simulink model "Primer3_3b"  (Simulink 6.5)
settings: Solver=ode23t  SolverMode=SingleTasking  StartTime=0.0  StopTime=1  RelTol=1e-3  AbsTol=1e-6
undefined symbols (not defined in the file or in its folder): Continuous, powergui, steady, ZData
libraries: powerlib x5, powerlib_extras x2

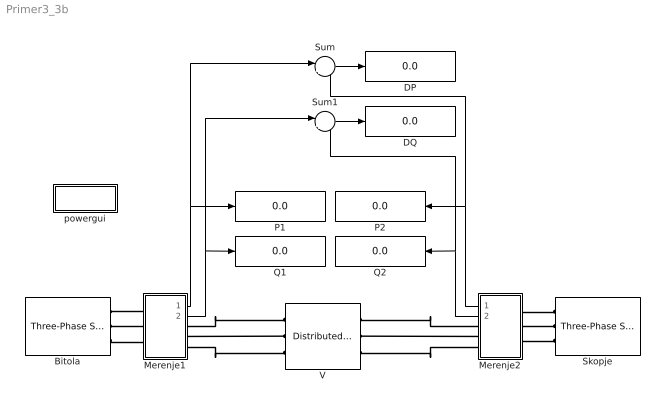
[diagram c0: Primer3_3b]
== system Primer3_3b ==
  Bitola : powerlib/Electrical Sources/Three-Phase Source  DialogController=PMDialogs.PMDefaultMaskDlg  SystemSampleTime=-1  Voltage=410e3  PhaseAngle=0  Frequency=50  InternalConnection=Yg  SpecifyImpedance=on  Resistance=0.8929  Inductance=16.58e-3  ShortCircuitLevel=sqrt(3)*400e3*16e3  BaseVoltage=400e3  XRratio=10
  DP : Display
  DQ : Display
  Merenje1 : Subsystem
  Merenje2 : Subsystem  Orientation=left
  P1 : Display
  P2 : Display
  Q1 : Display
  Q2 : Display
  Skopje : powerlib/Electrical Sources/Three-Phase Source  Orientation=left  DialogController=PMDialogs.PMDefaultMaskDlg  SystemSampleTime=-1  Voltage=395e3  PhaseAngle=-2.5  Frequency=50  InternalConnection=Yg  SpecifyImpedance=on  Resistance=0.8929  Inductance=16.58e-3  ShortCircuitLevel=sqrt(3)*400e3*14e3  BaseVoltage=400e3  XRratio=10
  Sum : Sum  Inputs=|++
  Sum1 : Sum  Inputs=|++
  V : powerlib/Elements/Distributed Parameters Line  DialogController=PMDialogs.PMDefaultMaskDlg  SystemSampleTime=-1  Phases=3  Frequency=50  Resistance=[0.029983 0.29405]  Inductance=[0.0010055 0.0025377]  Capacitance=[1.1784e-008 8.6541e-009]  Length=113.5  x1=[0 8.60953493752654e-011 155617.901806502 -377100.173822709;0.000106379256748321 8.65325079837872e-011 168131.358149619 -371689.815392539;0.000212758513496643 8.68730275722288e-011 180457.046333984 -365864.355859094;0.000319137770244964 8.7116527850222e-011 192581.201100092 -359630.30106294;0.000425517026993286 8.72627368780204e-011 204490.282259832 -352994.613161546;0.000531896283741607 8.7311491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  x2=[0 1.52828084545043e-010 143893.096531519 -373225.666404169;0.000106379256748321 1.57548911798779e-010 156283.637924653 -368209.241884694;0.000212758513496643 1.62093789310554e-010 168499.6426266 -362781.603346936;0.000319137770244964 1.66457641386629e-010 180527.467871754 -356948.812347202;0.000425517026993286 1.70635594501455e-010 192353.681052273 -350717.382913801;0.000531896283741607 1.7462298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  x3=[0 -7.90373299703389e-013 525.422105317868 -979.122392884629;0.000106379256748321 -7.55164225839465e-013 557.844919090553 -961.019300144194;0.000212758513496643 -7.19111788799262e-013 589.644734783168 -941.842946433889;0.000319137770244964 -6.82256251742466e-013 620.786038539719 -921.614747798094;0.000425517026993286 -6.44638774726363e-013 651.234051926655 -900.357294975707;0.000531896283741607 -6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  x4=[0 1.19047082254412e-012 334.073009196058 -1629.8040871509;0.000106379256748321 1.13114510037133e-012 388.344425208523 -1617.73135760439;0.000212758513496643 1.07055612168819e-012 442.182140342785 -1603.85195474176;0.000319137770244964 1.0087715519266e-012 495.52602894023 -1588.18137900235;0.000425517026993286 9.45860391747901e-013 548.316516844957 -1570.73713119736;0.000531896283741607 8.81892899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  x5=0.000531896283741607  Measurements=None
  powergui : Subsystem  AncestorBlock=powerlib/powergui  InitFcn=powergui( 'InitFcn_Callback' , gcb , 0 , [ ] );  mask(PSB option menu block){SimulationMode=Continuous, SampleTime=50e-6, echomessages=off, RestoreLinks=warning, x0status=steady, Frange=[0:2:500], Ylog=off, Xlog=on, ShowGrid=off, save=off, variable=ZData, structure=, ZoomFFT=on, StartTime=0.0, cycles=1, DisplayStyle=1, fundamental=60, FreqAxis=off, MaxFrequency=1000, frequencyindice=50, frequencyindicesteady=1, RmsSteady=2, display=off, Ts=0, frequency=60, methode=off, HookPort=off, Interpol=off}
      mask prompts: SimulationMode "Simulation mode"; SampleTime "Sample time Ts (when simulation mode is Discrete) (s)"; echomessages "Echo  Messages"; RestoreLinks "Restore disabled links"; x0status "Initial electrical states status"; Frange "Impedance tool: Frequency Range"; Ylog "Impedance tool: Log impedance"; Xlog "Impedance tool: log Frequency"; ShowGrid "Impedance tool: grid"; save "Impedance tool: Save Data To Workspace"; variable "Impedance tool: Variable Name"; structure "Structure Name (PSBFFTSCOPE)"; ZoomFFT "ZoomFFT (PSBFFTSCOPE)"; StartTime "Start Time (PSBFFTSCOPE)"; cycles "Cycles (PSBFFTSCOPE)"; DisplayStyle "Display style (PSBFFTSCOPE)"; fundamental "Fundamental (PSBFFTSCOPE)"; FreqAxis "Frequency Axis (PSBFFTSCOPE)"; MaxFrequency "Max Frequency (PSBFFTSCOPE)"; frequencyindice "Load flow frequency (Hz)"; frequencyindicesteady "Frequency indice (STEADYSTATE)"; RmsSteady "RMS display (STEADYSTATE)"; display "Display Results"; Ts "OBSOLETE 1"; frequency "Phasor frequency (Hz)"; methode "Phasor simulation"; HookPort "Hook port"; Interpol "Interpolate"
      mask init:
      | powerlibroot = which('powersysdomain');
      | PSBroot = powerlibroot(1:end-16);
      | %
      | switch SimulationMode
      | 	case 1
      | 		message=sprintf('Continuous');
      | 	case 2
      |         SampleTimeeval=evalin('base',SampleTime,'NaN');
      |         if isnan(SampleTimeeval)
      |             message=sprintf('Warning !!,\nUndefined sample time');
      |         else
      |             message=sprintf('Discrete,\nTs = %.4g s.',SampleTimeeval);
      |         end
      | 	case 3
      | 		message=sprintf('Phasors');
      | end
      | if strcmp(bdroot,'powerlib')
      |   message='powergui';
      | end
      | power_initmask();
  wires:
  Merenje1/1(P) -> P1/1, Sum/1
  Merenje1/2(Q) -> Q1/1, Sum1/1
  Merenje2/1(P) -> P2/1, Sum/2
  Merenje2/2(Q) -> Q2/1, Sum1/2
  Sum/1 -> DP/1
  Sum1/1 -> DQ/1
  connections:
  Bitola/RConn1 -- Merenje1/LConn1
  Bitola/RConn2 -- Merenje1/LConn2
  Bitola/RConn3 -- Merenje1/LConn3
  Merenje1/RConn2 -- V/LConn2
  Merenje1/RConn3 -- V/LConn3
  Merenje1/RConn1 -- V/LConn1
  Merenje2/LConn2 -- Skopje/RConn2
  Merenje2/LConn1 -- Skopje/RConn1
  Merenje2/LConn3 -- Skopje/RConn3
  V/RConn2 -- Merenje2/RConn2
  Merenje2/RConn3 -- V/RConn3
  Merenje2/RConn1 -- V/RConn1

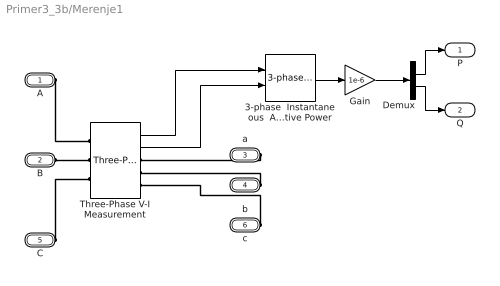
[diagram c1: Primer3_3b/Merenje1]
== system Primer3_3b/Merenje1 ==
  3-phase  Instantaneous  Active & Reactive Power : powerlib_extras/Measurements/3-phase  Instantaneous  Active & Reactive Power  DialogController=PMDialogs.PMDefaultMaskDlg  SystemSampleTime=-1
  Demux : Demux  Outputs=2
  Gain : Gain  Gain=1e-6
  Three-Phase V-I Measurement : powerlib/Measurements/Three-Phase V-I Measurement  DialogController=PMDialogs.PMDefaultMaskDlg  SystemSampleTime=-1  VoltageMeasurement=phase-to-ground  SetLabelV=off  LabelV=Vabc  Vpu=off  CurrentMeasurement=yes  SetLabelI=off  LabelI=Iabc  Ipu=off  Pbase=100e6  Vbase=500e3  OutputType=Complex  PhasorSimulation=off  PSBequivalent=0
  A : PMIOPort  Port=1  Side=Left
  B : PMIOPort  Port=2  Side=Left
  a : PMIOPort  Orientation=left  Port=3  Side=Right
  b : PMIOPort  Orientation=left  Port=4  Side=Right
  C : PMIOPort  Port=5  Side=Left
  c : PMIOPort  Orientation=left  Port=6  Side=Right
  P : Outport
  Q : Outport  Port=2
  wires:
  Three-Phase V-I Measurement/1 -> 3-phase  Instantaneous  Active & Reactive Power/1
  Three-Phase V-I Measurement/2 -> 3-phase  Instantaneous  Active & Reactive Power/2
  Demux/1 -> P/1
  Demux/2 -> Q/1
  3-phase  Instantaneous  Active & Reactive Power/1 -> Gain/1
  Gain/1 -> Demux/1
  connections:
  A/RConn1 -- Three-Phase V-I Measurement/LConn1
  B/RConn1 -- Three-Phase V-I Measurement/LConn2
  a/RConn1 -- Three-Phase V-I Measurement/RConn1
  b/RConn1 -- Three-Phase V-I Measurement/RConn2
  C/RConn1 -- Three-Phase V-I Measurement/LConn3
  c/RConn1 -- Three-Phase V-I Measurement/RConn3

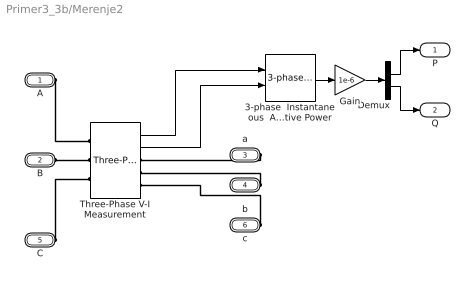
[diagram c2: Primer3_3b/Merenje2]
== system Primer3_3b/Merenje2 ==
  3-phase  Instantaneous  Active & Reactive Power : powerlib_extras/Measurements/3-phase  Instantaneous  Active & Reactive Power  DialogController=PMDialogs.PMDefaultMaskDlg  SystemSampleTime=-1
  Demux : Demux  Outputs=2
  Gain : Gain  Gain=1e-6
  Three-Phase V-I Measurement : powerlib/Measurements/Three-Phase V-I Measurement  DialogController=PMDialogs.PMDefaultMaskDlg  SystemSampleTime=-1  VoltageMeasurement=phase-to-ground  SetLabelV=off  LabelV=Vabc  Vpu=off  CurrentMeasurement=yes  SetLabelI=off  LabelI=Iabc  Ipu=off  Pbase=100e6  Vbase=500e3  OutputType=Complex  PhasorSimulation=off  PSBequivalent=0
  A : PMIOPort  Port=1  Side=Left
  B : PMIOPort  Port=2  Side=Left
  a : PMIOPort  Orientation=left  Port=3  Side=Right
  b : PMIOPort  Orientation=left  Port=4  Side=Right
  C : PMIOPort  Port=5  Side=Left
  c : PMIOPort  Orientation=left  Port=6  Side=Right
  P : Outport
  Q : Outport  Port=2
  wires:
  Demux/2 -> Q/1
  Demux/1 -> P/1
  Three-Phase V-I Measurement/2 -> 3-phase  Instantaneous  Active & Reactive Power/2
  Three-Phase V-I Measurement/1 -> 3-phase  Instantaneous  Active & Reactive Power/1
  3-phase  Instantaneous  Active & Reactive Power/1 -> Gain/1
  Gain/1 -> Demux/1
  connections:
  c/RConn1 -- Three-Phase V-I Measurement/RConn3
  C/RConn1 -- Three-Phase V-I Measurement/LConn3
  b/RConn1 -- Three-Phase V-I Measurement/RConn2
  a/RConn1 -- Three-Phase V-I Measurement/RConn1
  B/RConn1 -- Three-Phase V-I Measurement/LConn2
  A/RConn1 -- Three-Phase V-I Measurement/LConn1

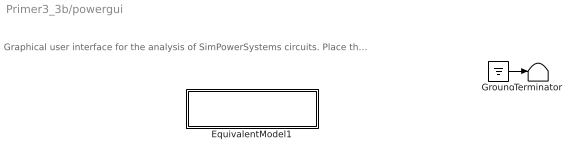
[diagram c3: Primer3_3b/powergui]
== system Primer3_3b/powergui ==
  note: Graphical user interface for the analysis of SimPowerSystems circuits. Place the Powergui block in the top-level of your model and double-click on it to open the GUI.
  EquivalentModel1 : Subsystem
  Ground : Ground
  Terminator : Terminator
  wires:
  Ground/1 -> Terminator/1

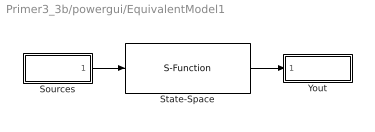
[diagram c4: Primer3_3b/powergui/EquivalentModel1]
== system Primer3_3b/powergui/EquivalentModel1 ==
  Sources : Subsystem
  State-Space : S-Function  FunctionName=sfun_spssw_contc  Parameters=A, B, C, D, x0
  Yout : Subsystem
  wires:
  State-Space/1 -> Yout/1(v,i)
  Sources/1(u) -> State-Space/1

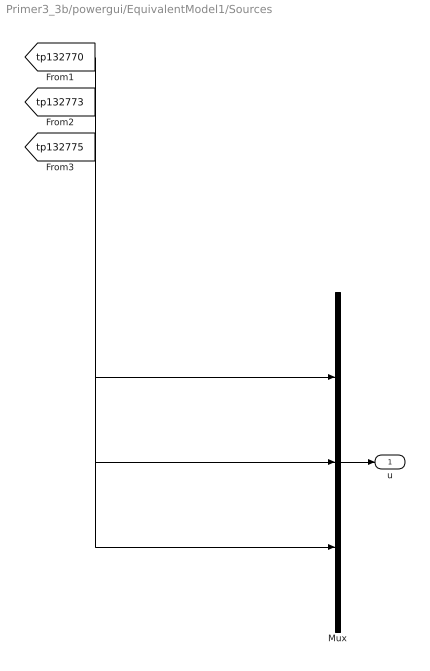
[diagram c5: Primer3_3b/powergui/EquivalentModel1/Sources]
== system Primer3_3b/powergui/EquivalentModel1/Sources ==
  Mux : Mux  Inputs=[6 3 3]
  u : Outport
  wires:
  Mux/1 -> u/1
  [tp132770] -> Mux/1
  [tp132773] -> Mux/2
  [tp132775] -> Mux/3

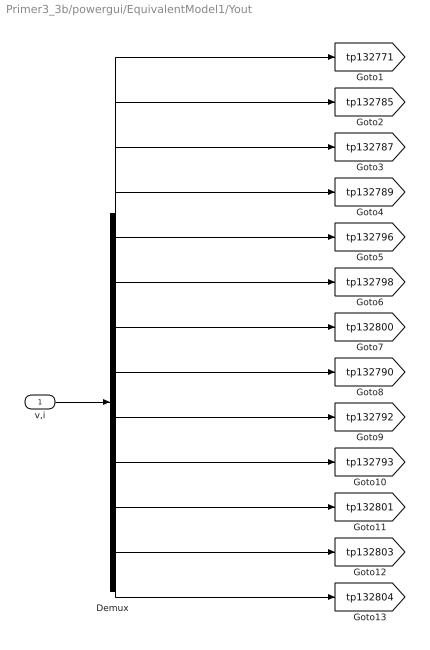
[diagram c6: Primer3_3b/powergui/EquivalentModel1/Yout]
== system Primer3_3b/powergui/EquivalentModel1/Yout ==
  v,i : Inport
  Demux : Demux  Outputs=[6 1 1 1 1 1 1 1 1 1 1 1 1]
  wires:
  v,i/1 -> Demux/1
  Demux/1 -> [tp132771]
  Demux/2 -> [tp132785]
  Demux/3 -> [tp132787]
  Demux/4 -> [tp132789]
  Demux/5 -> [tp132796]
  Demux/6 -> [tp132798]
  Demux/7 -> [tp132800]
  Demux/8 -> [tp132790]
  Demux/9 -> [tp132792]
  Demux/10 -> [tp132793]
  Demux/11 -> [tp132801]
  Demux/12 -> [tp132803]
  Demux/13 -> [tp132804]
